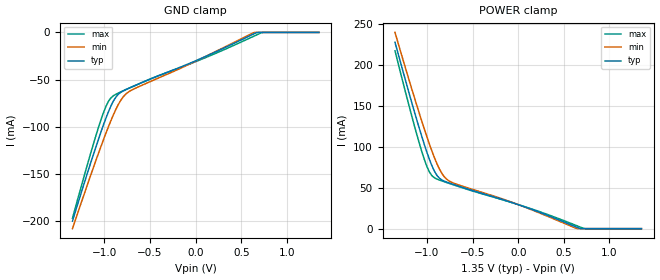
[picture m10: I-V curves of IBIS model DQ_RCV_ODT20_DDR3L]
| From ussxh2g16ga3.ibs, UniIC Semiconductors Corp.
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|   Model DQ_RCV_ODT20_DDR3L
[Model] DQ_RCV_ODT20_DDR3L
Model_type Input
Vinl =  0.540V
Vinh =  0.810V
C_comp   0.966pF   0.965pF   0.967pF
[Model Spec]
Vinh   0.810V   0.776V   0.860V
Vinl   0.540V   0.506V   0.590V
[Temperature Range]   25.000   95.000   -40.000
[Voltage Range]   1.350V   1.283V   1.450V
[GND_clamp]
|Voltage   I(typ)   I(min)   I(max)
-1.35V    -200.3mA   -208.3mA   -197.2mA
-1.098V   -122.9mA   -137.2mA   -111.1mA
-986mV    -91.68mA   -107.6mA   -79.12mA
-930mV    -78.37mA   -93.92mA   -69.63mA
-874mV    -68.58mA   -81.56mA   -65.65mA
-818mV    -63.41mA   -71.6mA    -63.05mA
-762mV    -60.54mA   -65.12mA   -60.59mA
-650mV    -55.77mA   -58.78mA   -55.79mA
22mV      -29.21mA   -29.52mA   -30.16mA
638mV     -1.516mA   -163.3uA   -3.995mA
750mV     0A         0A         0A
1.35V     0A         0A         0A
[POWER_clamp]
|Voltage   I(typ)   I(min)   I(max)
-1.35V    228mA      240mA      217.5mA
-1.114V   134.1mA    151.9mA    116.4mA
-1.002V   93.94mA    113mA      76.52mA
-946mV    77.08mA    95.1mA     64.89mA
-890mV    65.12mA    79.33mA    60.62mA
-834mV    59.4mA     67.17mA    58.3mA
-778mV    56.69mA    59.95mA    56.16mA
-666mV    52.5mA     53.98mA    51.97mA
62mV      27.02mA    26.78mA    27.23mA
650mV     1.352mA    0A         3.235mA
734mV     0A         0A         0A
1.35V     0A         0A         0A
